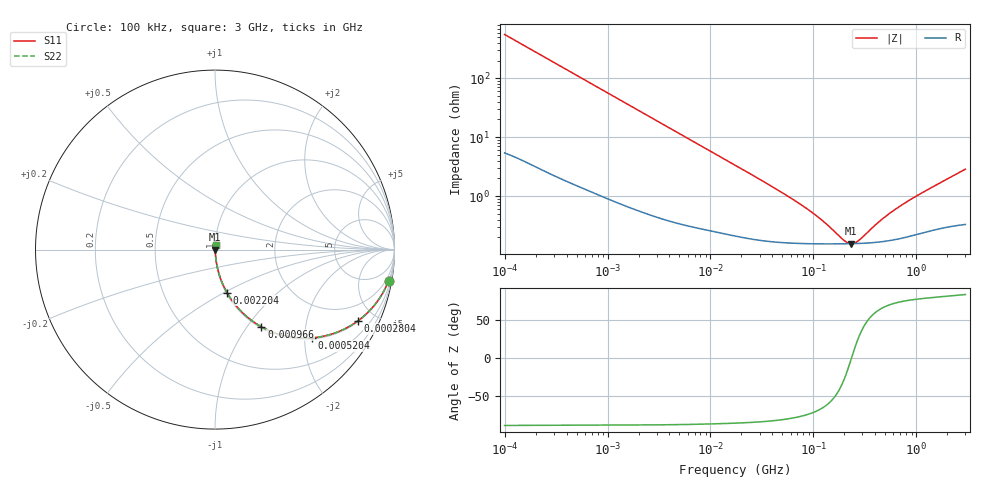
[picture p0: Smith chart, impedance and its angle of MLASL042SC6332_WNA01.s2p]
! MLASL042SC6332_WNA01  S-PARAMETER MODEL  ( Standard Model )
! Model Generated by TAIYO YUDEN Corporation (http://www.ty-top.com)
! Version 1.0
! TAIYO YUDEN Control No. 240524
! Copyright(c) 2024 TAIYO YUDEN CO.,LTD. All Rights Reserved.
! Product Description (link to TY-COMPAS)
! https://ds.yuden.co.jp/TYCOMPAS/or/detail?pn=MLASL042SC6332KWNA01&u=M
! Products Name : Multilayer Ceramic Capacitors
! Characteristics :
!  Capacitance : 3300 [pF] , Rated Voltage : 10 [V] , TCC : X6S
!  Case Size : 0.4 x 0.2 / 0.016 x 0.008 [mm/inch] , Thickness : 0.2 / 0.008 [mm/inch]
!  (Conditions: Temperature = 25 [degC] , DC Bias Voltage = 0 [V])
! External Node Assignments :
!  1  o---| |---o  2
! GND o---------o GND
! Frequency Range : 100kHz  -  3GHz  [ 401 STEP ]
# MHZ S RI R 50
! Freq[MHz].  S11 Real  S11 Imag  S21 Real  S21 Imag  S12 Real  S12 Imag  S22 Real  S22 Imag
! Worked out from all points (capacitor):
!   401 points, 100 kHz to 3 GHz, reference 50 ohm
!   read as one part in series: C = 2.86 nF near 105.3 kHz
!   lowest |Z| = 156 mohm at 233.9 MHz (marker M1)
!   series resonance near 235.3 MHz, so ESL is about 160 pH
!   S11 on the Smith chart (normalised r, x): 100 kHz: 1, -11; 280.4 kHz: 1.05, -3.99; 520.4 kHz: 1.03, -2.16; 966 kHz: 1.02, -1.17; 2.204 MHz: 1.01, -0.52; 3 GHz: 1.01, +0.06
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0.1  0.9671 -0.1737  0.0329 0.1737  0.0329 0.1737  0.9671 -0.1737
0.176296  0.9067 -0.2854  0.0933 0.2854  0.0933 0.2854  0.9067 -0.2854
0.280357  0.7968 -0.3965  0.2032 0.3965  0.2032 0.3965  0.7968 -0.3965
0.391939  0.6702 -0.4639  0.3298 0.4639  0.3298 0.4639  0.6702 -0.4639
0.520403  0.5383 -0.4918  0.4617 0.4918  0.4617 0.4918  0.5383 -0.4918
0.562235  0.5005 -0.4932  0.4995 0.4932  0.4995 0.4932  0.5005 -0.4932
0.965977  0.2584 -0.43  0.7416 0.43  0.7416 0.43  0.2584 -0.43
1.421866  0.1416 -0.34  0.8584 0.34  0.8584 0.34  0.1416 -0.34
2.203618  0.0669 -0.2398  0.9331 0.2398  0.9331 0.2398  0.0669 -0.2398
3.161081  0.0355 -0.1735  0.9645 0.1735  0.9645 0.1735  0.0355 -0.1735
6.848882  0.00989 -0.0829  0.9901 0.0829  0.9901 0.0829  0.00989 -0.0829
17.7727  0.00313 -0.0325  0.9969 0.0325  0.9969 0.0325  0.00313 -0.0325
51.12795  0.00174 -0.011  0.9983 0.011  0.9983 0.011  0.00174 -0.011
97.38194  0.00157 -0.00501  0.9984 0.00501  0.9984 0.00501  0.00157 -0.00501
132.6759  0.00155 -0.00303  0.9985 0.00303  0.9985 0.00303  0.00155 -0.00303
195.2919  0.00154 -0.000939  0.9985 0.000939  0.9985 0.000939  0.00154 -0.000939
233.9019  0.00155 -2.95e-05  0.9984 2.95e-05  0.9984 2.95e-05  0.00155 -2.95e-05
280.1453  0.00157 0.000879  0.9984 -0.000879  0.9984 -0.000879  0.00157 0.000879
412.3589  0.00165 0.00296  0.9984 -0.00296  0.9984 -0.00296  0.00165 0.00296
547.5153  0.00177 0.00472  0.9982 -0.00472  0.9982 -0.00472  0.00177 0.00472
1042.837  0.00236 0.0101  0.9976 -0.0101  0.9976 -0.0101  0.00236 0.0101
3000  0.00409 0.0283  0.9959 -0.0283  0.9959 -0.0283  0.00409 0.0283
